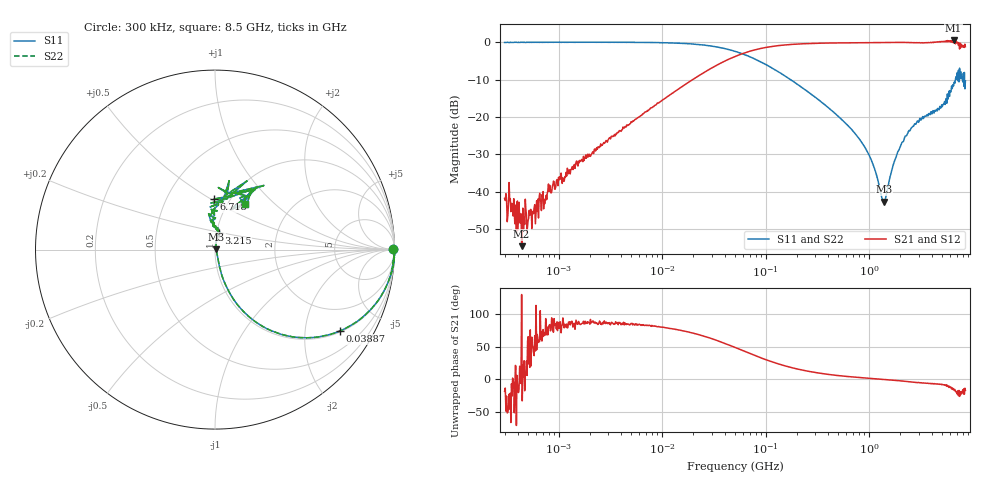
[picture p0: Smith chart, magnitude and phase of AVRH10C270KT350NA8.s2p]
! S-Parameter Data Generated by TDK Corporation
! Copyright(C) 2023 TDK Corporation.
! All Rights Reserved.
! TDK P/N: AVRH10C270KT350NA8 (Varistor)
! Property: V1mA=27V
! Size(LxWxT): 1x0.5x0.5mm
! Model Type: s2p (Touchstone File Format Version 1.0)
! Frequency: DC=Yes Start=0.3MHz Stop=8500MHz 802points Log-sweep
! Model Generated on Oct. 12, 2023
! Port Assignments:
!  1 ---N--- 2
! Applicable Conditions:
!  Temperature = 25 degC
!  DC Bias Voltage = 0 V
!  Small Signal Operation
! Terms and conditions regarding TDK Simulation Models
! (1)This simulation model is being provided solely for informational purposes. Please refer to the specifications of the products in terms of detailed characteristics of such products.
! (2)In no event shall TDK Corporation of any of its subsidiaries be liable for any loss or damage arising, directly or indirectly,
!  From any information contained in this simulation model, including, but not limited to loss or damages arising from any inaccuracies, omissions or errors in connection with such information.
! (3)Any and all copyrights on this simulation model are owned by TDK Corporation.
!  Duplication or redistribution of this simulation model without prior written permission from TDK Corporation is prohibited.
! (4)This simulation model is subject to any modification or change without any prior notice.
! (5)Neither TDK Corporation nor any of its subsidiaries shall make any warranty, express or implied,
!  Including but not limited to the correctness, implied warranties of merchantability and fitness for a particular purpose with respect to this simulation models.
! (6)The use of this simulation model shall be deemed to have consented to the terms and conditions hereof.
# Hz S MA R 50
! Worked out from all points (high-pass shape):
!   801 points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, 300 kHz to 8.5 GHz, reference 50 ohm
!   highest |S21| = 0.47 dB at 6.531 GHz (marker M1); lowest = -54.6 dB at 438.1 kHz (marker M2)
!   |S21| within 3 dB of the highest: 68 MHz to end of sweep
!   lowest |S11| = -42.7 dB at 1.392 GHz (marker M3), VSWR 1.01, Z = 50.7 + j0.154 ohm
!   |S11| at or under -10 dB: 173.7 MHz to 6.808 GHz (6.634 GHz wide, 190 % of centre); 7.172331 GHz to 7.198796 GHz (26.46 MHz wide, 0.368 % of centre); 8.353 GHz to end of sweep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
!   |S22| runs from -42.7 to 0.0 dB; largest |S21 - S12| = 0
!   S11 on the Smith chart (normalised r, x): 300 kHz: open; 38.87 MHz: 1.04, -3.04; 3.215 GHz: 1.02, +0.19; 6.718 GHz: 0.84, +0.51; 8.5 GHz: 1.19, +0.67
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300000  0.9923 0.1  0.008114 -18.4  0.008114 -18.4  0.9923 0.1
349513  0.9931 0.0  0.006954 -6.7  0.006954 -6.7  0.9931 0.0
438095  1.001 -0.1  0.001863 130.1  0.001863 130.1  1.001 -0.1
1667335  0.9983 -1.5  0.02697 85.7  0.02697 85.7  0.9983 -1.5
9160262  0.9875 -8.8  0.153 80.9  0.153 80.9  0.9875 -8.8
2.076269e7  0.9399 -19.3  0.3307 70.0  0.3307 70.0  0.9399 -19.3
3.886999e7  0.8304 -33.1  0.5455 56.1  0.5455 56.1  0.8304 -33.1
5.049752e7  0.7551 -40.1  0.6439 49.0  0.6439 49.0  0.7551 -40.1
1.203782e8  0.4358 -62.2  0.8852 25.8  0.8852 25.8  0.4358 -62.2
2.804659e8  0.1977 -73.6  0.9631 11.4  0.9631 11.4  0.1977 -73.6
8.428256e8  0.04613 -71.4  0.9863 2.5  0.9863 2.5  0.04613 -71.4
1.06509e9  0.02497 -64.4  0.9894 1.3  0.9894 1.3  0.02497 -64.4
1.391719e9  0.007309 12.0  0.9929 -0.1  0.9929 -0.1  0.007309 12.0
1.542892e9  0.01324 62.8  0.994 -0.7  0.994 -0.7  0.01324 62.8
1.735053e9  0.02455 77.1  0.9948 -1.4  0.9948 -1.4  0.02455 77.1
2.125542e9  0.04643 80.0  0.993 -2.6  0.993 -2.6  0.04643 80.0
3.215129e9  0.09386 77.7  0.9843 -5.3  0.9843 -5.3  0.09386 77.7
5.149026e9  0.1457 95.7  1.025 -8.1  1.025 -8.1  0.1457 95.7
6.530872e9  0.2603 95.1  1.055 -14.2  1.055 -14.2  0.2603 95.1
6.718408e9  0.2812 91.5  1.046 -15.6  1.046 -15.6  0.2812 91.5
7.468552e9  0.4494 52.7  0.8107 -26.2  0.8107 -26.2  0.4494 52.7
8.5e9  0.3027 57.1  0.8733 -16.9  0.8733 -16.9  0.3027 57.1
